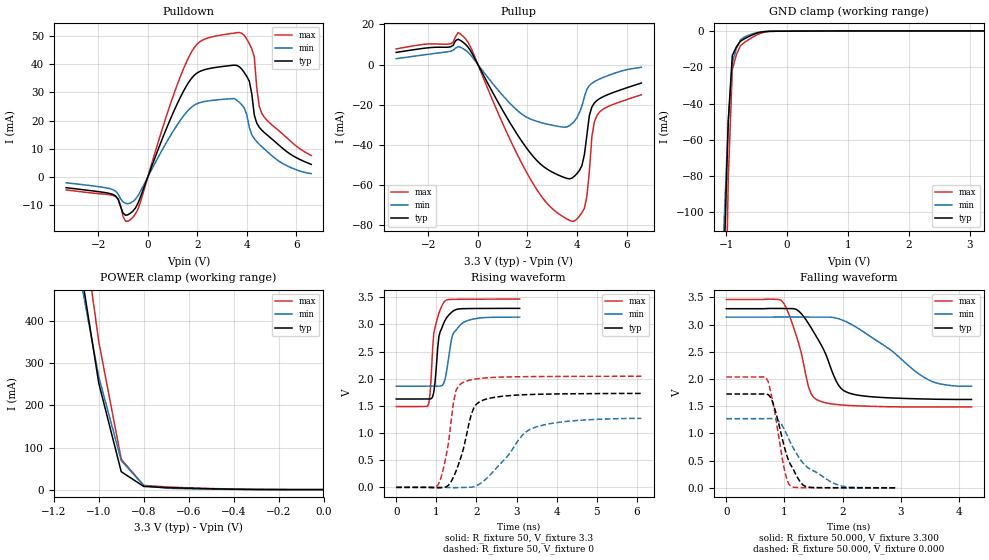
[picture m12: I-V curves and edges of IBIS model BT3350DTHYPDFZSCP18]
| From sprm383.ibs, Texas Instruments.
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|   Model Cell BT3350DTHYPDFZSCP18
[Model]   BT3350DTHYPDFZSCP18
Model_type   I/O
Polarity   Non-Inverting
Enable   Active-Low
Vinl =  0.8V
Vinh =  2V
Cref =  15.0000pF
Rref =  100.0000M
Vref =  0V
Vmeas =  1.65
C_comp   1.493p   1.456463p   1.529415p
[Model Spec]
Vinl   0.8V   0.8V   0.8V
Vinh   2V   2V   2V
[Temperature Range]   25   105   0
[Voltage Range]   3.3   3.14   3.47
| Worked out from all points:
|   slope of the pulldown table from 0 to 0.495 V, typ, clamps not added: 42.9 ohm
|   slope of the pullup table from 0 to 0.495 V, typ, clamps not added: 42.8 ohm
|   GND clamp passes 1 mA (typ) near -0.49 V on its own axis
|   POWER clamp passes 1 mA (typ) near -0.40 V on its own axis
|   rising waveform, R_fixture 50, V_fixture 3.3: 20-80 % time 180ps typ, 223ps min, 153ps max; typ from 1.63 V to 3.3 V
|   rising waveform, R_fixture 50, V_fixture 0: 20-80 % time 379ps typ, 853ps min, 252ps max; typ from 0 V to 1.73 V
|   falling waveform, R_fixture 50.000, V_fixture 3.300: 20-80 % time 444ps typ, 941ps min, 289ps max; typ from 3.29 V to 1.62 V
|   falling waveform, R_fixture 50.000, V_fixture 0.000: 20-80 % time 296ps typ, 568ps min, 196ps max; typ from 1.73 V to 0.001 V
[POWER_clamp]
|   voltage   I(typ)   I(min)   I(max)
-3.3V     9.96A      8.611A     10.94A
-1.067V   478.9mA    459.2mA    610.8mA
-1.033V   365.9mA    363.6mA    481.1mA
-1V       253mA      268mA      351.4mA
-900mV    42.61mA    69.08mA    72.31mA
-800mV    7.612mA    9.647mA    10.2mA
-700mV    4.877mA    3.434mA    6.369mA
-600mV    3.319mA    2.085mA    4.366mA
-300mV    394.6uA    184.3uA    564.2uA
-11.55fV  142.7uA    86.75uA    197.1uA
[Pulldown]
|   voltage   I(typ)   I(min)   I(max)
-3.3V     -3.798mA   -2.054mA   -4.568mA
-1.3V     -6.728mA   -5.045mA   -6.952mA
-700mV    -12.84mA   -9.217mA   -15.12mA
-400mV    -9.372mA   -6.707mA   -11.45mA
900mV     20.28mA    14.47mA    25.55mA
1.8V      35.39mA    25.05mA    44.9mA
3.6V      39.59mA    27.18mA    51.23mA
4.1V      33.99mA    17.52mA    47.31mA
4.3V      22.03mA    13.6mA     42.63mA
4.4V      19.11mA    12.56mA    31.7mA
4.6V      16.65mA    10.8mA     22.67mA
6.6V      4.483mA    1.197mA    7.628mA
[Pullup]
|   voltage   I(typ)   I(min)   I(max)
-3.3V     6.066mA    2.957mA    7.802mA
-600mV    11.14mA    7.958mA    14.14mA
1.3V      -29.12mA   -19.42mA   -37.44mA
2.2V      -45.34mA   -27.53mA   -58.77mA
2.9V      -52.9mA    -29.98mA   -70.61mA
3.8V      -56.58mA   -29.42mA   -78.12mA
4.3V      -44.86mA   -15.96mA   -71.63mA
4.4V      -35.19mA   -12.35mA   -65.67mA
4.5V      -25.37mA   -10.47mA   -53.29mA
4.6V      -21.19mA   -9.34mA    -36.14mA
4.8V      -17.96mA   -7.847mA   -25.51mA
6.6V      -9.2mA     -1.379mA   -15.05mA
[GND_clamp]
|   voltage   I(typ)   I(min)   I(max)
-3.3V     -13.48A    -11.6A     -14.64A
-1.1V     -237.7mA   -179.8mA   -391.2mA
-1.033V   -124.4mA   -104mA     -204.7mA
-966.7mV  -49.64mA   -49.89mA   -81.4mA
-900mV    -13.39mA   -17.29mA   -21.13mA
-833.3mV  -8.667mA   -9.512mA   -12.97mA
-766.7mV  -5.587mA   -4.821mA   -7.994mA
-700mV    -4.155mA   -3.217mA   -6.204mA
-500mV    -1.116mA   -794.3uA   -2.088mA
-300mV    -91.68uA   -71.35uA   -179.9uA
3.233V    142.6uA    88.12uA    196.8uA
[Ramp]
| variable   typ   min   max
dV/dt_f   1.028903/0.4459997n  0.8144917/1.009357n   1.205632/0.2895588n
dV/dt_r   1.04764/0.3796482n  0.7898414/0.9077102n   1.234582/0.2484465n
R_load = 50
[Rising Waveform]
R_fixture = 50
V_fixture = 3.3
V_fixture_min = 3.14
V_fixture_max = 3.47
|   time   V(typ)   V(min)   V(max)
0s        1.627V     1.863V     1.488V
780ps     1.627V     1.864V     1.493V
844ps     1.628V     1.864V     1.729V
936ps     1.751V     1.864V     2.833V
968ps     1.936V     1.864V     2.946V
1.064ns   2.778V     1.864V     3.207V
1.22ns    3.079V     2V         3.436V
1.408ns   3.241V     2.811V     3.461V
1.628ns   3.289V     3.011V     3.464V
3.076ns   3.296V     3.134V     3.466V
[Rising Waveform]
R_fixture = 50
V_fixture = 0
V_fixture_min = 0
V_fixture_max = 0
|   time   V(typ)   V(min)   V(max)
0s        45.65uV    21.44uV    77.14uV
1.056ns   -9.459mV   -1.046uV   62.16mV
1.24ns    6.56mV     -1.637mV   563mV
1.428ns   189.5mV    -7.204mV   1.572V
1.492ns   301.3mV    -5.978mV   1.786V
1.676ns   711mV      -1.558mV   1.935V
1.928ns   1.454V     9.535mV    1.989V
2.24ns    1.625V     156.1mV    2.016V
3.42ns    1.711V     1.095V     2.039V
6.108ns   1.729V     1.269V     2.046V
[Falling Waveform]
R_fixture = 50.000
V_fixture = 3.300
V_fixture_min = 3.140
V_fixture_max = 3.470
|  time   V(typ)   V(min)   V(max)
0s        3.293V     3.138V     3.462V
944ps     3.297V     3.14V      3.449V
1.028ns   3.295V     3.141V     3.314V
1.2ns     3.282V     3.14V      2.814V
1.416ns   3.017V     3.139V     1.851V
1.588ns   2.712V     3.138V     1.604V
1.932ns   1.886V     3.109V     1.529V
2.104ns   1.746V     3.032V     1.515V
3.484ns   1.632V     1.984V     1.487V
4.22ns    1.625V     1.867V     1.487V
[Falling Waveform]
R_fixture = 50.000
V_fixture = 0.000
V_fixture_min = 0.000
V_fixture_max = 0.000
|  time   V(typ)   V(min)   V(max)
0s        1.725V     1.272V     2.038V
684ps     1.725V     1.272V     2.023V
744ps     1.691V     1.274V     1.855V
804ps     1.555V     1.269V     1.554V
984ps     813mV      1.104V     414.5mV
1.044ns   586.1mV    969.8mV    153.3mV
1.104ns   429.5mV    832.2mV    34.02mV
1.344ns   36.13mV    428.2mV    3.711mV
1.884ns   2.814mV    69.25mV    998.6uV
2.944ns   1.163mV    3.17mV     268.8uV
